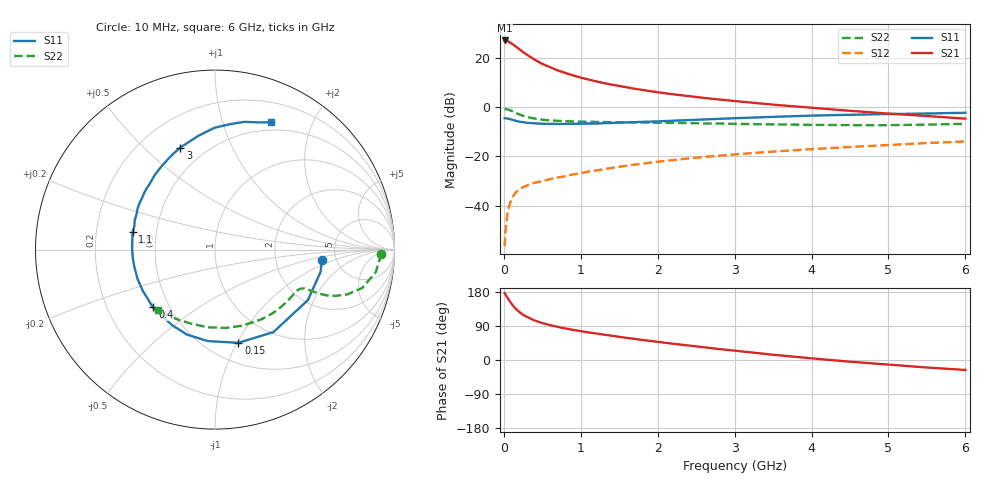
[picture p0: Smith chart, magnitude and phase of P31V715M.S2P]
! SIEMENS Small Signal Semiconductors
! BFP181
! Si NPN RF Bipolar Junction Transistor in SOT143
! VCE = 1.75 V  IC = 15 mA
! Common Emitter S-Parameters:  March  1996
# GHz  S  MA  R  50
!  f  S11  S21  S12  S22
! GHz  MAG  ANG  MAG  ANG  MAG  ANG  MAG  ANG
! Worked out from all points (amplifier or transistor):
!   36 points, 10 MHz to 6 GHz, reference 50 ohm
!   highest |S21| = 27.2 dB at 10 MHz (marker M1)
!   |S21| within 3 dB of that: start of sweep to 178.8 MHz
!   unconditionally stable (mu >= 1): start of sweep to 14.49 MHz; 476.6 MHz to end of sweep
!   at 250 MHz: K = 0.64, MSG = 27.5 dB, |S12| = -32.5 dB
!   at 1.4 GHz: K = 1.54, MAG = 12.6 dB, |S12| = -24.7 dB
!   at 6 GHz: K = 1.21, MAG = 1.9 dB, |S12| = -13.9 dB
!   S11 on the Smith chart (normalised r, x): 10 MHz: 3.83, -0.72; 150 MHz: 0.70, -1.01; 400 MHz: 0.41, -0.34; 1.1 GHz: 0.36, +0.09; 3 GHz: 0.37, +0.65; 6 GHz: 0.41, +1.45
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0.01  0.5984 -5.8  22.91 176.5  0.0015 76.7  0.9267 -1.4
0.02  0.6014 -11.8  22.83 173.4  0.0029 86.8  0.9205 -3.1
0.05  0.5892 -28.5  22.23 163.1  0.0079 78.0  0.9043 -8.0
0.1  0.5632 -54.6  19.96 148.4  0.0138 65.1  0.8478 -14.6
0.15  0.5354 -75.9  17.56 136.3  0.0183 58.3  0.7784 -18.7
0.2  0.5113 -94.4  15.3 126.9  0.0215 54.7  0.7195 -21.0
0.25  0.4987 -108.2  13.28 119.3  0.0238 51.4  0.672 -22.3
0.3  0.4841 -119.6  11.74 113.8  0.0257 50.0  0.6378 -22.8
0.4  0.4721 -137.1  9.334 104.3  0.0292 48.5  0.5897 -23.2
0.5  0.4632 -150.4  7.648 97.5  0.0316 48.0  0.5599 -23.3
0.6  0.4612 -159.5  6.554 92.1  0.0346 49.3  0.5421 -23.5
0.7  0.4595 -168.0  5.627 87.4  0.0373 50.7  0.5308 -24.1
0.9  0.4615 179.1  4.463 79.7  0.0434 51.6  0.5164 -25.5
1.1  0.4691 167.8  3.677 72.8  0.0495 52.8  0.5079 -27.7
1.5  0.4886 151.9  2.717 61.0  0.0619 53.4  0.498 -32.9
1.8  0.5064 140.8  2.258 52.9  0.0712 53.1  0.4915 -37.6
2.2  0.5341 129.0  1.842 42.9  0.0844 51.3  0.4827 -44.3
3  0.6006 108.8  1.343 24.7  0.1102 46.4  0.4609 -59.6
3.5  0.6399 98.5  1.134 13.9  0.1259 43.0  0.4501 -70.6
4.5  0.7044 83.1  0.85 -4.5  0.1561 35.1  0.4345 -95.3
5.5  0.7483 71.3  0.665 -19.8  0.1879 27.2  0.4453 -120.7
6  0.7755 66.2  0.589 -26.3  0.2025 22.5  0.4626 -133.0
